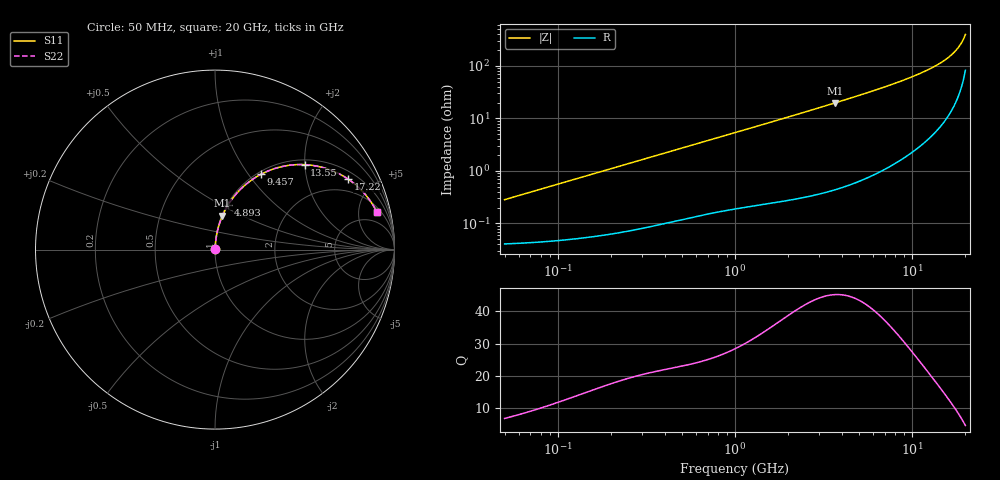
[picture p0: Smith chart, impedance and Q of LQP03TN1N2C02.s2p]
!Murata Part Number: LQP03TN1N2C02
!These Parameters are Measured in Series Mode Connection
!  o--[Z]--o
!Port1  Port2
!  o-------o
!Freq. Start=50[MHz] Stop=20[GHz], 401[Steps]
# Hz S RI R 50
!Freq.(Hz) S11(Real) S11(Imag) S21(Real) S21(Imag) S12(Real) S12(Imag) S22(Real) S22(Imag)
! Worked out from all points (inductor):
!   401 points, 50 MHz to 20 GHz, reference 50 ohm
!   read as one part in series: L = 893 pH near 51.52 MHz
!   highest Q = 45.1 at 3.681 GHz (marker M1), where L = 856 pH
!   S11 on the Smith chart (normalised r, x): 50 MHz: 1.00, +0.01; 4.893 GHz: 1.01, +0.53; 9.457 GHz: 1.04, +1.15; 13.55 GHz: 1.11, +2.00; 17.22 GHz: 1.34, +3.57; 20 GHz: 2.64, +7.76
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5e7  0.000416 0.00281  0.9996 -0.00281  0.9996 -0.00281  0.000416 0.00281
1.364002e8  0.000583 0.00759  0.9994 -0.00759  0.9994 -0.00759  0.000583 0.00759
3.721004e8  0.00136 0.0203  0.9986 -0.0203  0.9986 -0.0203  0.00136 0.0203
1e9  0.00473 0.0532  0.9953 -0.0532  0.9953 -0.0532  0.00473 0.0532
1.714689e9  0.0107 0.0901  0.9893 -0.0901  0.9893 -0.0901  0.0107 0.0901
2.728004e9  0.0239 0.1416  0.9761 -0.1416  0.9761 -0.1416  0.0239 0.1416
3.680849e9  0.0416 0.1889  0.9584 -0.1889  0.9584 -0.1889  0.0416 0.1889
4.89267e9  0.0715 0.2465  0.9285 -0.2465  0.9285 -0.2465  0.0715 0.2465
6.125241e9  0.1104 0.3011  0.8896 -0.3011  0.8896 -0.3011  0.1104 0.3011
7.442007e9  0.1611 0.3538  0.8389 -0.3538  0.8389 -0.3538  0.1611 0.3538
8.389408e9  0.2031 0.3872  0.7969 -0.3872  0.7969 -0.3872  0.2031 0.3872
9.457416e9  0.2559 0.4195  0.7441 -0.4195  0.7441 -0.4195  0.2559 0.4195
1.131968e10  0.3599 0.4594  0.6401 -0.4594  0.6401 -0.4594  0.3599 0.4594
1.354865e10  0.5 0.4733  0.5 -0.4733  0.5 -0.4733  0.5 0.4733
1.460232e10  0.5698 0.4646  0.4302 -0.4646  0.4302 -0.4646  0.5698 0.4646
1.550395e10  0.6301 0.4483  0.3699 -0.4483  0.3699 -0.4483  0.6301 0.4483
1.646126e10  0.6937 0.4212  0.3063 -0.4212  0.3063 -0.4212  0.6937 0.4212
1.721783e10  0.7429 0.392  0.2571 -0.392  0.2571 -0.392  0.7429 0.392
1.800918e10  0.7924 0.3532  0.2076 -0.3532  0.2076 -0.3532  0.7924 0.3532
1.855685e10  0.8251 0.3211  0.1749 -0.3211  0.1749 -0.3211  0.8251 0.3211
1.940974e10  0.8721 0.261  0.1279 -0.261  0.1279 -0.261  0.8721 0.261
2e10  0.9009 0.2111  0.0991 -0.2111  0.0991 -0.2111  0.9009 0.2111
